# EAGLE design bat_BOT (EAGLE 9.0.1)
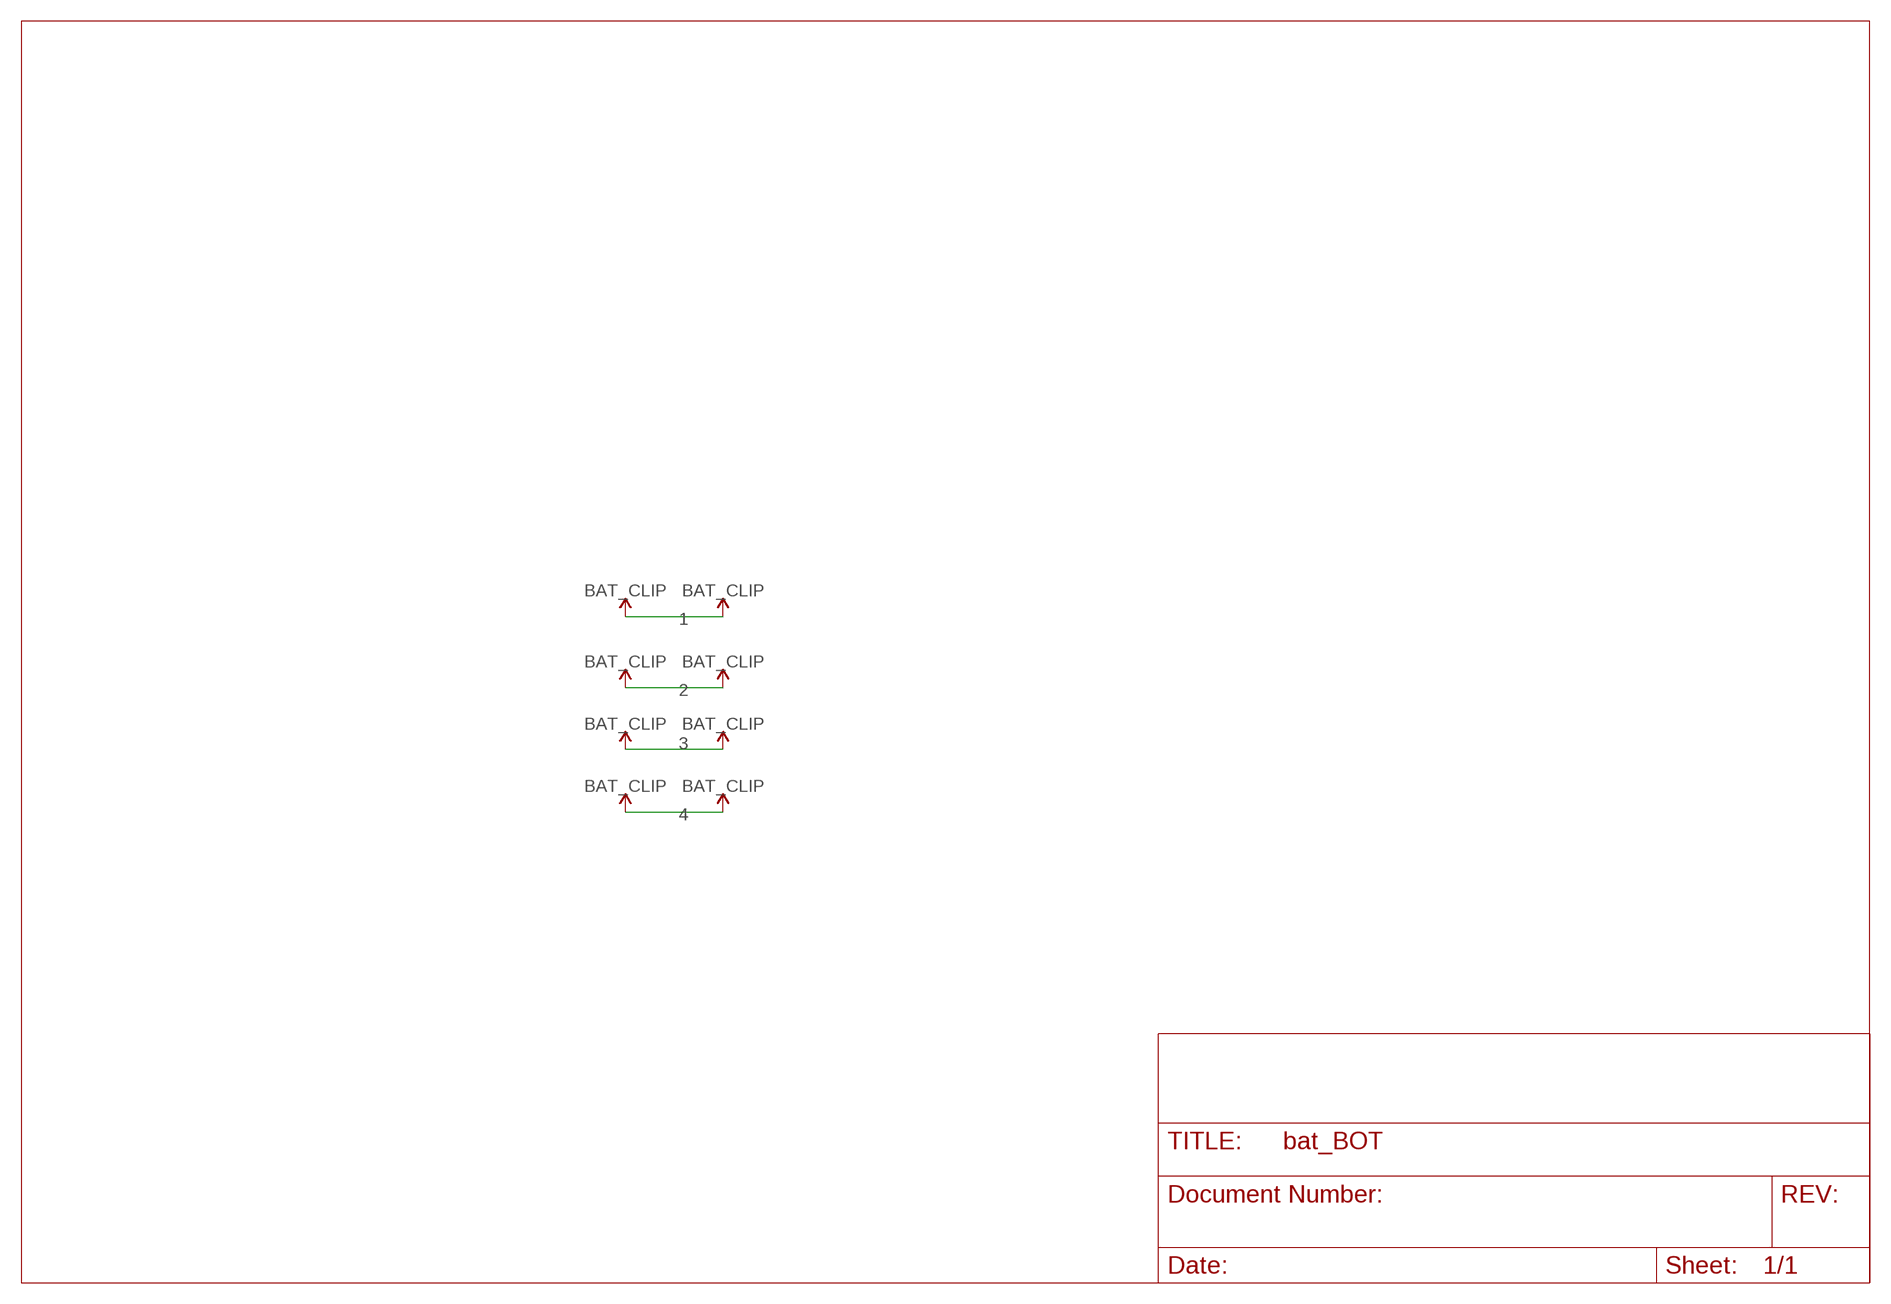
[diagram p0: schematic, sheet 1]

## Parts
U$1  BAT_CLIP  [CLIP]
U$2  BAT_CLIP  [CLIP]
U$3  BAT_CLIP  [CLIP]
U$4  BAT_CLIP  [CLIP]
U$5  BAT_CLIP  [CLIP]
U$6  BAT_CLIP  [CLIP]
U$7  BAT_CLIP  [CLIP]
U$8  BAT_CLIP  [CLIP]

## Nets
1: U$1.P$1(V_BATT) U$1.P$2(V_BATT) U$1.P$3(V_BATT) U$1.P$4(V_BATT) U$2.P$1(V_BATT) U$2.P$2(V_BATT) U$2.P$3(V_BATT) U$2.P$4(V_BATT)
2: U$3.P$1(V_BATT) U$3.P$2(V_BATT) U$3.P$3(V_BATT) U$3.P$4(V_BATT) U$6.P$1(V_BATT) U$6.P$2(V_BATT) U$6.P$3(V_BATT) U$6.P$4(V_BATT)
3: U$4.P$1(V_BATT) U$4.P$2(V_BATT) U$4.P$3(V_BATT) U$4.P$4(V_BATT) U$8.P$1(V_BATT) U$8.P$2(V_BATT) U$8.P$3(V_BATT) U$8.P$4(V_BATT)
4: U$5.P$1(V_BATT) U$5.P$2(V_BATT) U$5.P$3(V_BATT) U$5.P$4(V_BATT) U$7.P$1(V_BATT) U$7.P$2(V_BATT) U$7.P$3(V_BATT) U$7.P$4(V_BATT)

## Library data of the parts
U$1-U$8 = bat:BAT_CLIP

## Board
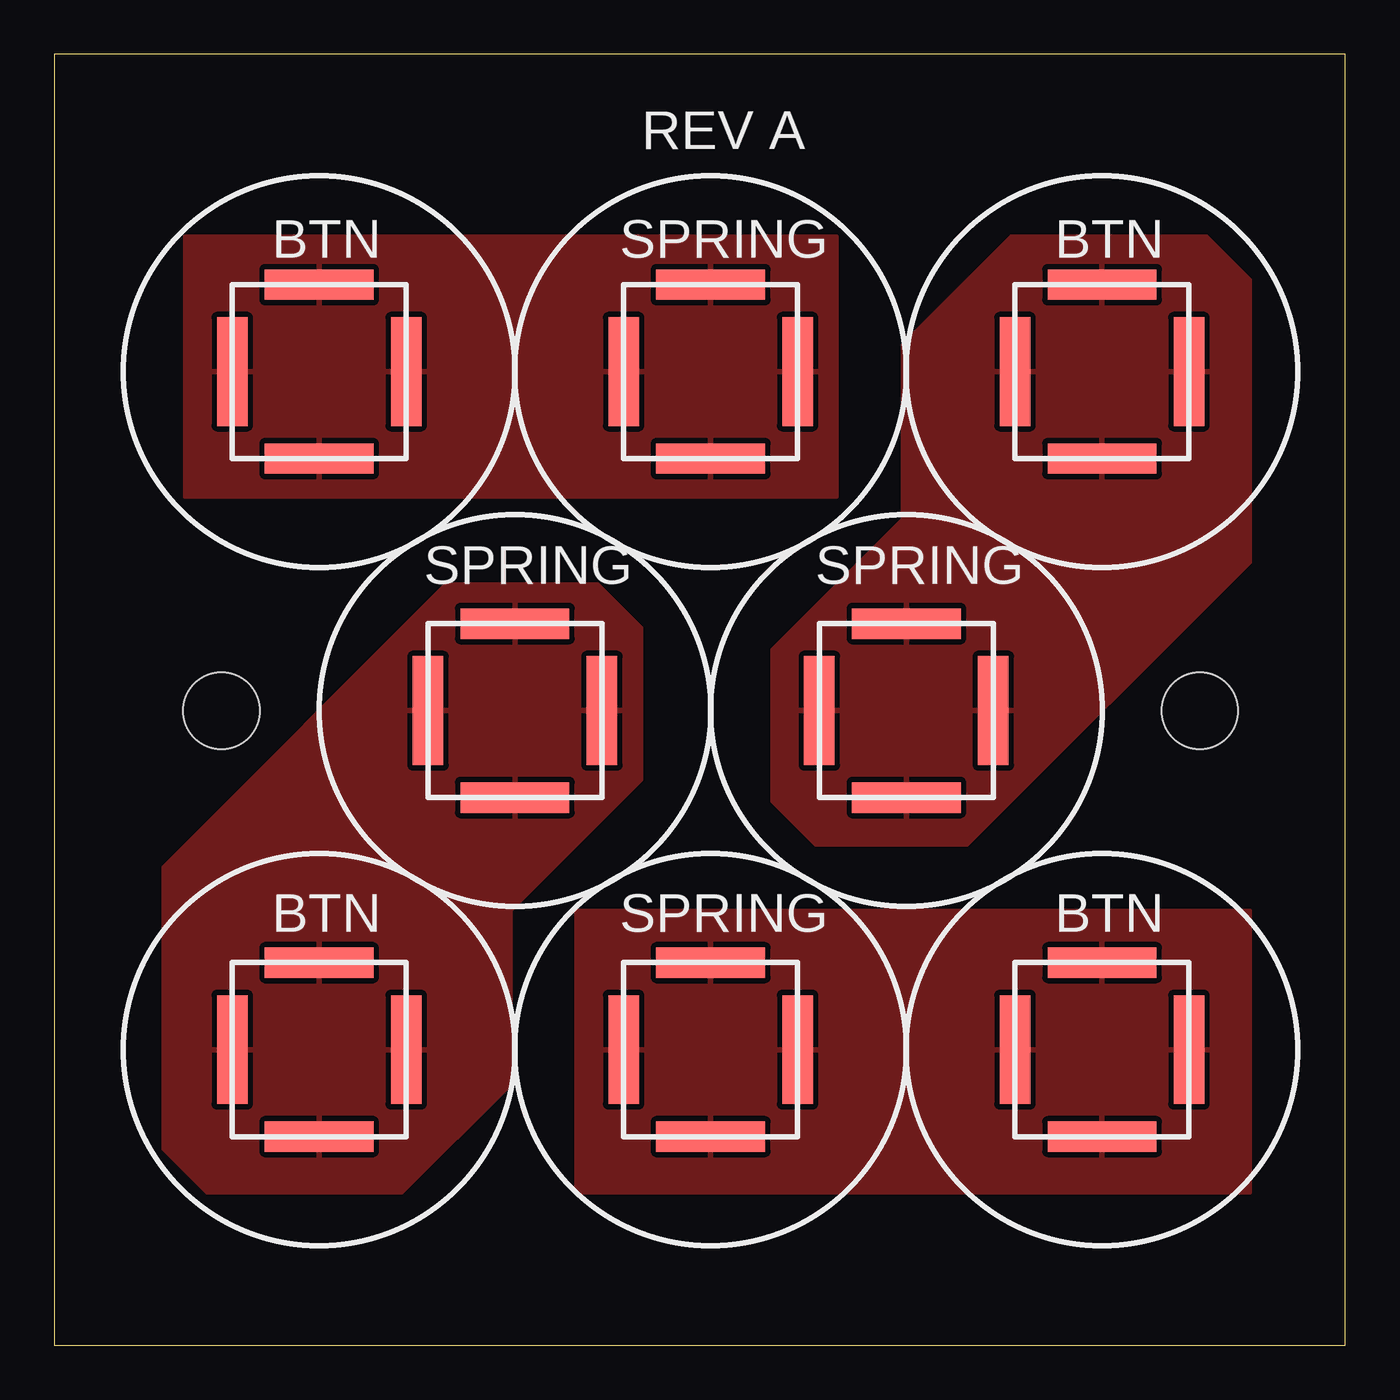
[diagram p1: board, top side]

Size 59.36 x 59.36 mm. Coordinates in mm from the lower left corner, seen from the top.
Outline: 0,0 59.36,0 59.36,59.36 0,59.36 0,0
Copper layers (1*16): Top 0.035mm / dielectric 1.5mm / Bottom 0.035mm
Design rules "default": minimum track width 6mil, minimum drill 0.35mm, track to track 6mil, track to pad 6mil, pad to pad 6mil, via to via 6mil, smd to smd 6mil, copper to edge 40mil, drill to drill 6mil, minimum pad ring 10mil, minimum via ring 8mil, stop-mask expansion 4mil, vias tented up to drill 0mil, thermal gap 10mil
Holes 3.5 mm at 7.68,29.18 52.68,29.18

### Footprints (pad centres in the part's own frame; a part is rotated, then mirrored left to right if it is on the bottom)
CLIP = smd 1.4 x 5: P$1 -4,0; P$2 4,0 | smd 5 x 1.4: P$3 0,4; P$4 0,-4

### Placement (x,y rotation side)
U$1  21.18,29.18 0 top
U$2  12.18,13.59 0 top
U$3  39.18,29.18 0 top
U$4  30.18,13.59 0 top
U$5  12.18,44.77 0 top
U$6  48.18,44.77 0 top
U$7  30.18,44.77 0 top
U$8  48.18,13.59 0 top

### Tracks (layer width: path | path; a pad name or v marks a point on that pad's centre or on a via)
1
  pour Top: 18,35 5,22 5,9 7,7 16,7 21,12 21,20 27,26 27,33 25,35
2
  pour Top: 42,23 55,36 55,49 53,51 44,51 39,46 39,38 33,32 33,25 35,23
3
  pour Top: 25,20 55,20 55,9 55,7 25,7 24,7 24,20
4
  pour Top: 36,51 6,51 6,39 36,39

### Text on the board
tPlace: REV A | BTN | SPRING | BTN | SPRING | SPRING | BTN | SPRING | BTN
